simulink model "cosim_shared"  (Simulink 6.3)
settings: Solver=ode45  StartTime=0.0  StopTime=1000  RelTol=1e-3
undefined symbols (not defined in the file or in its folder): cosim_xrc4_top, netlist_xrc4
libraries: adcosim_example_lib x1

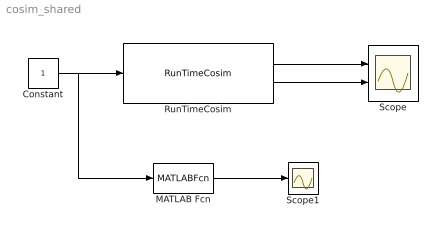
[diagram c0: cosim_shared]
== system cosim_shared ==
  Constant : Constant
  MATLAB Fcn : MATLABFcn  MATLABFcn=read_adregs
  RunTimeCosim : adcosim_example_lib/RunTimeCosim  index=0  bitstream=netlist_xrc4/cosim_xrc4_top.bit  freq=120  single_step=on  shared=Matlab
  Scope : Scope  NumInputPorts=2
  Scope1 : Scope
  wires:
  Constant/1 -> RunTimeCosim/1, MATLAB Fcn/1
  RunTimeCosim/1 -> Scope/1
  RunTimeCosim/2 -> Scope/2
  MATLAB Fcn/1 -> Scope1/1
